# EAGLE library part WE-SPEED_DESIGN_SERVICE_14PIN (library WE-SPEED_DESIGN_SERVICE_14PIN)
WE-Speedy Design Service, 14 Pin - Any application that fits package style - Switch Mode Power: Flyback, Forward, Push-Pull, Coupled Inductor -- Telecom Applications: xDSL, POTS Splitter Inductors
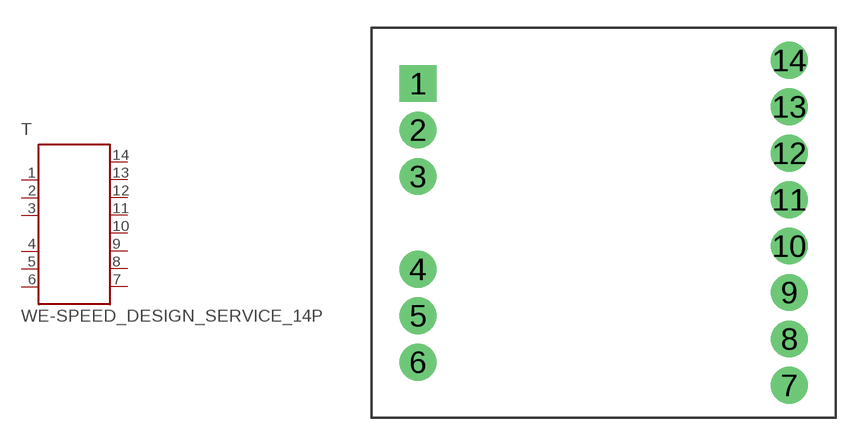
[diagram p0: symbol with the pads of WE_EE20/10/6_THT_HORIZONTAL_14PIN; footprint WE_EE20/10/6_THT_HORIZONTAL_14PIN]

Designator prefix T

## WE-SPEED_DESIGN_SERVICE_14PIN-750311911_EE20/10/6_THT (MPN: 750311911; OC_FARNELL: 1895750; OC_NEWARK: 47T5868; PACKAGE: EE20/10/6; SUPPLIER: Würth Elektronik eiSos GmbH)  [WE_EE20/10/6_THT_HORIZONTAL_14PIN]
1  1  pas
2  2  pas
3  3  pas
4  4  pas
5  5  pas
6  6  pas
7  7  pas
8  8  pas
9  9  pas
10  10  pas
11  11  pas
12  12  pas
13  13  pas
14  14  pas

## Footprint WE_EE20/10/6_THT_HORIZONTAL_14PIN (pad centres in mm)
Transformer, EE20/10/6 THT Horizontal 14 Pin
drill 1.32 square: 1 -10,7.5
drill 1.32: 2 -10,5; 3 -10,2.5; 4 -10,-2.5; 5 -10,-5; 6 -10,-7.5; 7 10,-8.75; 8 10,-6.25; 9 10,-3.75; 10 10,-1.25; 11 10,1.25; 12 10,3.75; 13 10,6.25; 14 10,8.75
